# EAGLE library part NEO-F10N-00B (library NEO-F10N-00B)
GNSS / GPS Modules u-blox F10 GNSS module Flash, TCXO, SAW, LNA LCC, 12x16 mm, 250 pcs/reel Source: Datasheet
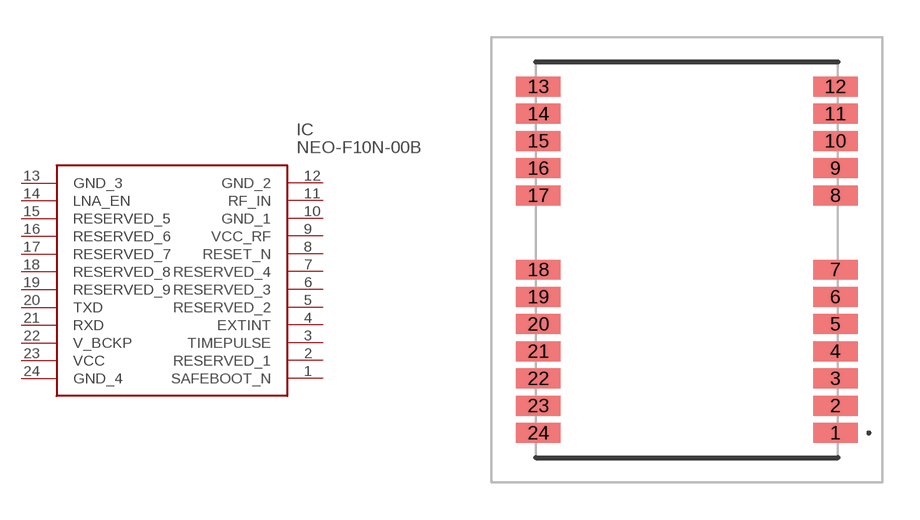
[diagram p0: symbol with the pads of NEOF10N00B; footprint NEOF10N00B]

Designator prefix IC

## NEO-F10N-00B (Arrow_Part_Number: NEO-F10N-00B; Arrow_Price-Stock: https://www.arrow.com/en/products/neo-f10n-00b/u-blox?utm_currency=USD&region=nac; Description: GNSS / GPS Modules u-blox F10 GNSS module Flash, TCXO, SAW, LNA LCC, 12x16 mm, 250 pcs/reel; Height: 2.6mm; Manufacturer_Name: u-blox; Manufacturer_Part_Number: NEO-F10N-00B; Mouser_Part_Number: 377-NEO-F10N-00B; Mouser_Price-Stock: https://www.mouser.co.uk/ProductDetail/u-blox/NEO-F10N-00B?qs=Imq1NPwxi76uVH%2FItRhLgw%3D%3D)  [NEOF10N00B]
1  SAFEBOOT_N
2  RESERVED_1
3  TIMEPULSE
4  EXTINT
5  RESERVED_2
6  RESERVED_3
7  RESERVED_4
8  RESET_N
9  VCC_RF
10  GND_1
11  RF_IN
12  GND_2
13  GND_3
14  LNA_EN
15  RESERVED_5
16  RESERVED_6
17  RESERVED_7
18  RESERVED_8
19  RESERVED_9
20  TXD
21  RXD
22  V_BCKP
23  VCC
24  GND_4

## Footprint NEOF10N00B (pad centres in mm)
NEO-F10N-00B-4
smd 1.8 x 0.8: 1 6,-7; 2 6,-5.9; 3 6,-4.8; 4 6,-3.7; 5 6,-2.6; 6 6,-1.5; 7 6,-0.4; 8 6,2.6; 9 6,3.7; 10 6,4.8; 11 6,5.9; 12 6,7; 13 -6,7; 14 -6,5.9; 15 -6,4.8; 16 -6,3.7; 17 -6,2.6; 18 -6,-0.4; 19 -6,-1.5; 20 -6,-2.6; 21 -6,-3.7; 22 -6,-4.8; 23 -6,-5.9; 24 -6,-7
